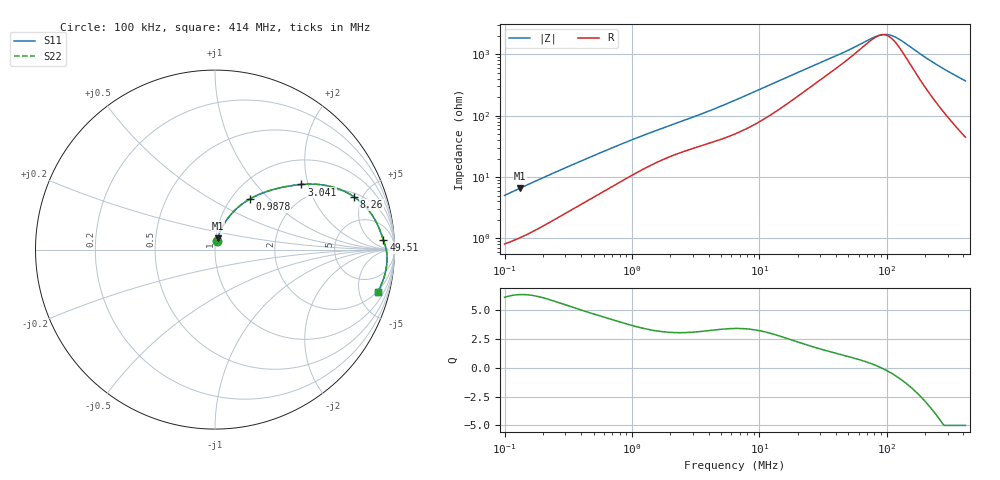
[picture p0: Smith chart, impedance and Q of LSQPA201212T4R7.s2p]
! LSQPA201212T4R7  S-PARAMETER MODEL  ( General Type )
! Model Generated by TAIYO YUDEN Corporation (http://www.ty-top.com)
! Version 2.0
! TAIYO YUDEN Control No. 100810NF25SB-FKC
! Copyright(c) 2007 TAIYO YUDEN CO.,LTD. All Rights Reserved.
! Product Description (link to TY-COMPAS)
! https://ds.yuden.co.jp/TYCOMPAS/or/detail?pn=LSQPA201212T4R7M&u=M
! Products Name : Inductors
! Characteristics :
!  Inductance : 4.7 uH , SRF(min) : 45 MHz , DC Resistance(max) : 0.65 Ohm
!  Rated Current : Saturation :360 mA , Temp Rise : 520 mA (40 degC)
!  Case Size : 2.0 x 1.25 / 0.079 x 0.049 [mm/inch] , Thickness : 1.25 / 0.049 [mm/inch]
!  (Conditions: Temperature = 25 degC , DC Bias Current/Voltage = 0A / 0V)
! External Node Assignments :
!  1  o---GGG---o  2
! GND o---------o GND
! Frequency Range : 0.1MHz  -  413.982163MHz  [ 402 STEP ]
# MHz S RI R 50
! Freq[MHz].  S11 Real  S11 Imag  S21 Real  S21 Imag  S12 Real  S12 Imag  S22 Real  S22 Imag
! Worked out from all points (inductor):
!   401 points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, 100 kHz to 414 MHz, reference 50 ohm
!   read as one part in series: L = 7.83 uH near 104.3 kHz
!   highest Q = 6.33 at 131.1 kHz (marker M1), where L = 7.82 uH
!   self-resonance near 89.9 MHz
!   S11 on the Smith chart (normalised r, x): 100 kHz: 1.02, +0.10; 987.8 kHz: 1.21, +0.77; 3.041 MHz: 1.59, +1.81; 8.26 MHz: 2.28, +4.28; 49.51 MHz: 18, +16; 414 MHz: 1.89, -7.30
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0.1  0.0105 0.0487  0.9895 -0.0487  0.9895 -0.0487  0.0105 0.0487
0.131085  0.0141 0.0629  0.9859 -0.0629  0.9859 -0.0629  0.0141 0.0629
0.244808  0.0321 0.1098  0.9679 -0.1098  0.9679 -0.1098  0.0321 0.1098
0.403501  0.0636 0.1634  0.9364 -0.1634  0.9364 -0.1634  0.0636 0.1634
0.637938  0.1156 0.2238  0.8844 -0.2238  0.8844 -0.2238  0.1156 0.2238
0.987802  0.1937 0.2818  0.8063 -0.2818  0.8063 -0.2818  0.1937 0.2818
1.628129  0.3113 0.3308  0.6887 -0.3308  0.6887 -0.3308  0.3113 0.3308
3.040622  0.4812 0.3629  0.5188 -0.3629  0.5188 -0.3629  0.4812 0.3629
4.516158  0.6025 0.3599  0.3975 -0.3599  0.3975 -0.3599  0.6025 0.3599
6.434145  0.7094 0.33  0.2906 -0.33  0.2906 -0.33  0.7094 0.33
8.260385  0.7741 0.2945  0.2259 -0.2945  0.2259 -0.2945  0.7741 0.2945
13.9015  0.8655 0.2063  0.1345 -0.2063  0.1345 -0.2063  0.8655 0.2063
25.96183  0.9149 0.1172  0.0851 -0.1172  0.0851 -0.1172  0.9149 0.1172
49.50526  0.9385 0.0535  0.0615 -0.0535  0.0615 -0.0535  0.9385 0.0535
83.31298  0.9521 0.00735  0.0479 -0.00735  0.0479 -0.00735  0.9521 0.00735
94.399  0.9546 -0.00483  0.0454 0.00483  0.0454 0.00483  0.9546 -0.00483
104.7562  0.9563 -0.0155  0.0437 0.0155  0.0437 0.0155  0.9563 -0.0155
113.8543  0.9574 -0.0245  0.0426 0.0245  0.0426 0.0245  0.9574 -0.0245
126.3461  0.9583 -0.0363  0.0417 0.0363  0.0417 0.0363  0.9583 -0.0363
195.638  0.9554 -0.0943  0.0446 0.0943  0.0446 0.0943  0.9554 -0.0943
256.4515  0.9463 -0.1386  0.0537 0.1386  0.0537 0.1386  0.9463 -0.1386
413.9822  0.9063 -0.2368  0.0937 0.2368  0.0937 0.2368  0.9063 -0.2368
